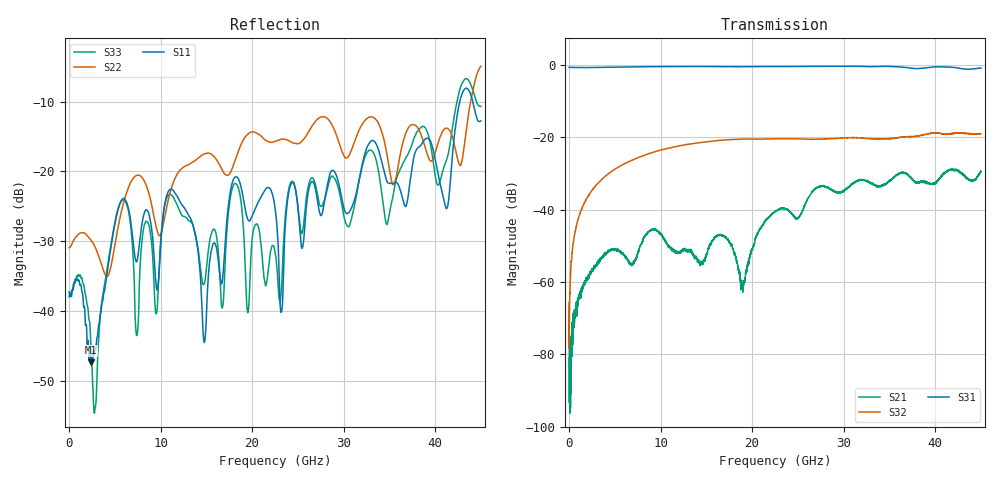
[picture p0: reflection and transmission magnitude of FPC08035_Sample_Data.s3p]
# MHz S DB R 50.00000
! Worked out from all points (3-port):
!   4500 points, 10 MHz to 45 GHz, reference 50 ohm
!   strongest paths, dB at 10 MHz, 11.26 GHz, 22.51 GHz, 33.76 GHz, 45 GHz:
!     S31: -0.7, -0.5, -0.5, -0.5, -0.9
!     S32: -65.7, -22.8, -20.5, -20.4, -19.1
!     S21: -71.7, -51.5, -40.6, -33.6, -29.4
!   lowest |S11| = -47.3 dB at 2.38 GHz (marker M1), VSWR 1.01, Z = 50.4 + j0.172 ohm
!   |S11| at or under -10 dB: start of sweep to 42.69 GHz; 44.11 GHz to end of sweep
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10  -37.22 138.2  -78.15 -33.8  -0.73 -0.6
    -71.70 -43.5  -30.93 7.7  -61.45 53.2
    -0.69 -0.7  -65.71 -58.7  -37.97 139.1
2380  -47.29 23.3  -57.40 94.3  -0.76 -12.9
      -57.14 94.5  -29.80 12.7  -35.16 79.8
      -0.74 -12.9  -35.17 80.2  -44.62 26.4
5840  -23.94 -115.5  -51.83 59.6  -0.63 -32.2
      -51.97 59.2  -25.08 -59.9  -27.64 64.4
      -0.62 -32.1  -27.64 64.3  -24.11 -128.3
7410  -32.88 -41.2  -52.87 100.9  -0.55 -41.5
      -53.00 102.9  -20.55 -31.5  -25.79 56.6
      -0.54 -41.4  -25.80 56.7  -43.49 -36.6
10920  -22.73 -155.4  -50.04 41.1  -0.50 -62.7
       -50.01 41.0  -23.66 -83.4  -23.01 37.9
       -0.48 -62.7  -23.01 37.9  -23.33 -145.0
14790  -44.46 -53.1  -54.20 86.2  -0.47 -86.3
       -54.04 87.5  -17.48 -79.6  -21.34 16.1
       -0.45 -86.3  -21.35 16.3  -36.05 -109.2
18020  -20.97 -170.1  -51.67 -12.0  -0.54 -106.6
       -51.78 -9.3  -18.87 -119.4  -20.63 -4.4
       -0.52 -106.6  -20.63 -4.3  -21.80 137.6
22510  -25.26 87.1  -40.47 141.0  -0.49 -133.9
       -40.55 140.9  -15.69 -131.1  -20.46 -35.7
       -0.46 -133.9  -20.46 -35.5  -31.51 122.4
23190  -40.15 10.5  -39.65 128.6  -0.49 -138.5
       -39.68 128.7  -15.38 -135.6  -20.42 -41.0
       -0.47 -138.5  -20.43 -40.9  -37.08 -1.0
45000  -12.77 -93.7  -29.62 -3.8  -0.89 66.4
       -29.37 -3.2  -4.93 -62.5  -19.11 137.2
       -0.87 66.9  -19.06 137.2  -10.68 -86.9
